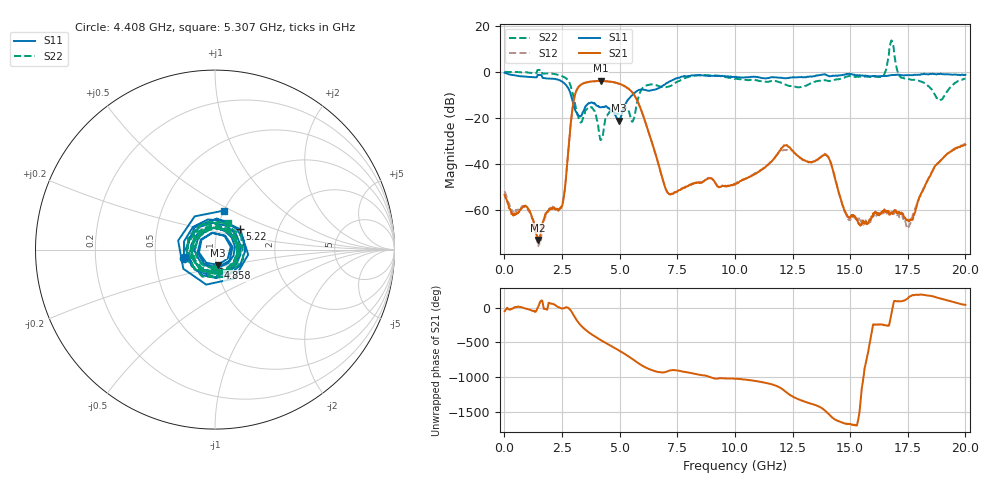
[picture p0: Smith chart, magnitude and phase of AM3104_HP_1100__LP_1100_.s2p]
!Created with skrf (http://scikit-rf.org).
# Hz S RI R 50.0
!freq ReS11 ImS11 ReS21 ImS21 ReS12 ImS12 ReS22 ImS22
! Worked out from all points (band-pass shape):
!   1601 points, 10 MHz to 20 GHz, reference 50 ohm
!   highest |S21| = -3.91 dB at 4.183 GHz (marker M1); lowest = -73.0 dB at 1.459 GHz (marker M2)
!   |S21| within 3 dB of the highest: 3.194 GHz to 5.325 GHz (2.131 GHz wide, 50 % of centre)
!   lowest |S11| = -21.3 dB at 4.958 GHz (marker M3), VSWR 1.19, Z = 51 - j8.71 ohm
!   |S11| at or under -10 dB: 2.885 GHz to 5.567 GHz (2.682 GHz wide, 63.5 % of centre)
!   |S22| runs from -29.6 to 13.6 dB; largest |S21 - S12| = 0.058
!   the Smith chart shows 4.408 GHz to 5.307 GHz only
!   S11 on the Smith chart (normalised r, x): 4.408 GHz: 0.70, -0.07; 4.858 GHz: 1.01, -0.21; 5.22 GHz: 1.29, +0.30; 5.307 GHz: 1.01, +0.46
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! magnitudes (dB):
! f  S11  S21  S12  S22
! 10 MHz  -0.4  -53.3  -51.7  0.0
! 1.459 GHz  -1.3  -73.0  -75.4  0.8
! 2.509 GHz  -4.3  -58.0  -57.3  -1.9
! 2.996 GHz  -14.2  -13.1  -13.2  -10.9
! 3.346 GHz  -19.0  -5.4  -5.5  -21.8
! 4.183 GHz  -15.5  -3.9  -3.9  -29.6
! 4.408 GHz  -14.9  -4.2  -4.2  -19.4
! 4.858 GHz  -19.8  -4.8  -4.9  -18.2
! 4.958 GHz  -21.3  -5.1  -5.2  -18.3
! 5.22 GHz  -14.9  -6.3  -6.3  -15.6
! 5.307 GHz  -13.0  -6.8  -6.8  -15.7
! 6.682 GHz  -7.2  -40.0  -40.0  -6.1
! 7.194 GHz  -4.1  -53.2  -53.2  -6.2
! 10.01 GHz  -2.4  -49.0  -48.5  -3.1
! 12.18 GHz  -2.8  -31.9  -33.9  -5.5
! 13.34 GHz  -2.1  -39.2  -39.3  -4.9
! 14.02 GHz  -1.6  -36.6  -36.4  -3.9
! 14.97 GHz  -0.9  -63.1  -64.4  -1.9
! 16.68 GHz  -1.6  -61.1  -60.8  7.2
! 17.53 GHz  -1.4  -64.8  -67.2  -3.0
! 18.9 GHz  -0.9  -38.8  -38.9  -12.3
! 20 GHz  -1.3  -31.7  -31.2  -3.0
